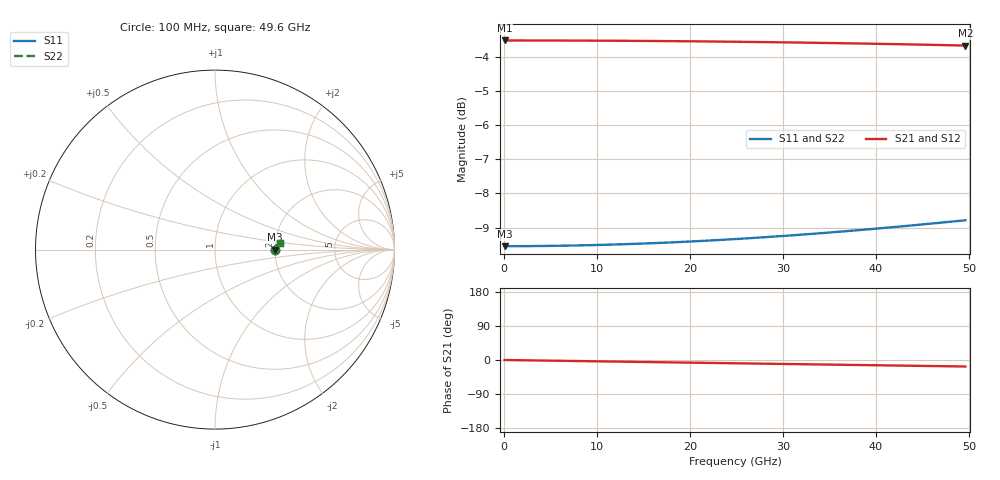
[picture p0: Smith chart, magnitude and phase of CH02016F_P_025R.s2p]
# GHz S RI R 25
! S-Parameters data
! Freq  reS11  imS11  reS21  imS21  reS12  imS12  reS22  imS22
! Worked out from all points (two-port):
!   100 points, 100 MHz to 49.6 GHz, reference 25 ohm
!   highest |S21| = -3.52 dB at 100 MHz (marker M1); lowest = -3.7 dB at 49.6 GHz (marker M2)
!   |S21| within 3 dB of the highest: start of sweep to end of sweep
!   lowest |S11| = -9.5 dB at 100 MHz (marker M3), VSWR 2.00, Z = 50 + j0.0102 ohm
!   |S11| at or under -10 dB: nowhere
!   |S22| runs from -9.5 to -8.8 dB; largest |S21 - S12| = 0
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0.1  0.3333 9.08e-05  0.6667 -0.000405  0.6667 -0.000405  0.3333 9.08e-05
2.1  0.3334 0.00191  0.6666 -0.0085  0.6666 -0.0085  0.3334 0.00191
4.1  0.3335 0.00372  0.6664 -0.0166  0.6664 -0.0166  0.3335 0.00372
6.1  0.3338 0.00552  0.666 -0.0247  0.666 -0.0247  0.3338 0.00552
8.6  0.3342 0.00777  0.6654 -0.0348  0.6654 -0.0348  0.3342 0.00777
10.6  0.3347 0.00955  0.6648 -0.0428  0.6648 -0.0428  0.3347 0.00955
12.6  0.3352 0.0113  0.664 -0.0509  0.664 -0.0509  0.3352 0.0113
14.6  0.3359 0.0131  0.663 -0.0589  0.663 -0.0589  0.3359 0.0131
16.6  0.3366 0.0148  0.662 -0.0669  0.662 -0.0669  0.3366 0.0148
18.6  0.3375 0.0165  0.6608 -0.0749  0.6608 -0.0749  0.3375 0.0165
20.6  0.3384 0.0182  0.6595 -0.0828  0.6595 -0.0828  0.3384 0.0182
22.6  0.3395 0.0199  0.658 -0.0908  0.658 -0.0908  0.3395 0.0199
25.1  0.3409 0.0219  0.656 -0.1006  0.656 -0.1006  0.3409 0.0219
27.1  0.3421 0.0235  0.6543 -0.1084  0.6543 -0.1084  0.3421 0.0235
29.1  0.3434 0.025  0.6524 -0.1162  0.6524 -0.1162  0.3434 0.025
31.1  0.3448 0.0265  0.6504 -0.124  0.6504 -0.124  0.3448 0.0265
33.1  0.3463 0.028  0.6483 -0.1317  0.6483 -0.1317  0.3463 0.028
37.1  0.3495 0.0308  0.6437 -0.147  0.6437 -0.147  0.3495 0.0308
39.1  0.3513 0.0321  0.6412 -0.1545  0.6412 -0.1545  0.3513 0.0321
41.6  0.3536 0.0337  0.6379 -0.1639  0.6379 -0.1639  0.3536 0.0337
45.6  0.3575 0.0361  0.6323 -0.1786  0.6323 -0.1786  0.3575 0.0361
49.6  0.3617 0.0383  0.6262 -0.1931  0.6262 -0.1931  0.3617 0.0383
